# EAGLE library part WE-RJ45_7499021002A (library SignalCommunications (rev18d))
WE-RJ45 LAN Transformer Order Code 7499021002A Design THT xBase-T 10/100 Base-T Ports 1x2 Application Standard Tab Position DOWN LED (Left-Right) NO EMI Fingers No Details see: http://katalog.we-online.de/en/pbs/WE-LAN-RJ45 Created by Yingchun Shan 2016 (C) Wurth Elektronik
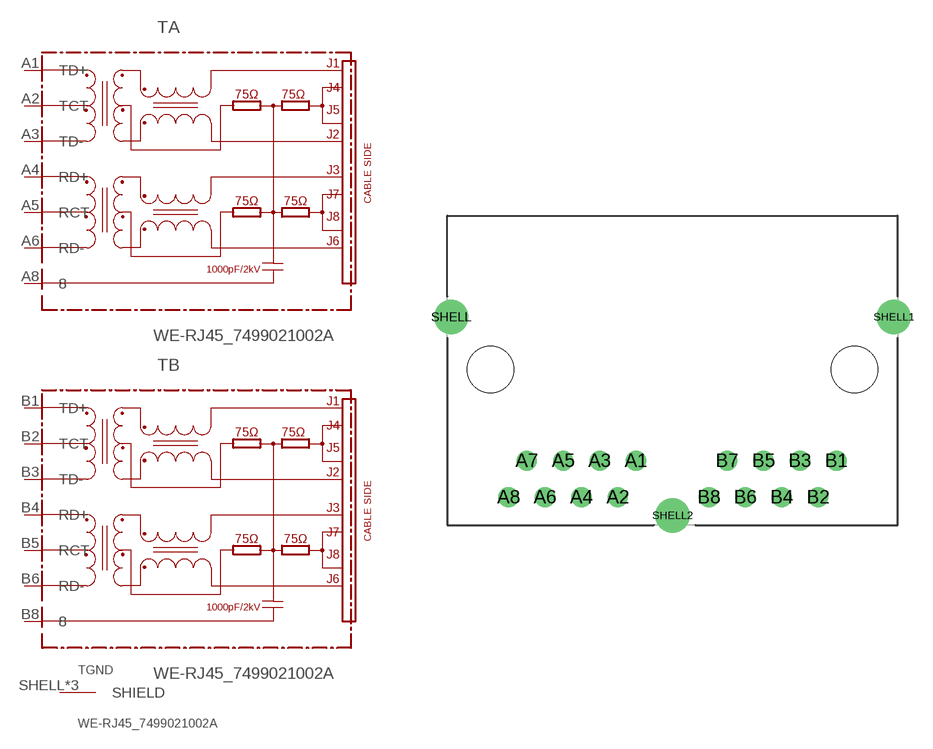
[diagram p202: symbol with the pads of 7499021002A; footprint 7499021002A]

Designator prefix T; gates A=7499021002A B=7499021002A GND=SHIELD

## WE-RJ45_7499021002A  [7499021002A]
A1  A:TD+
A2  A:TCT
A3  A:TD-
A4  A:RD+
A5  A:RCT
A6  A:RD-
A8  A:8
B1  B:TD+
B2  B:TCT
B3  B:TD-
B4  B:RD+
B5  B:RCT
B6  B:RD-
B8  B:8
SHELL  GND:SHIELD  pas
SHELL1  GND:SHIELD  pas
SHELL2  GND:SHIELD  pas

## Footprint 7499021002A (pad centres in mm)
drill 0.9: A1 -2.54,-6.35; A2 -3.81,-8.89; A3 -5.08,-6.35; A4 -6.35,-8.89; A5 -7.62,-6.35; A6 -8.89,-8.89; A7 -10.16,-6.35; A8 -11.43,-8.89; B1 11.43,-6.35; B2 10.16,-8.89; B3 8.89,-6.35; B4 7.62,-8.89; B5 6.35,-6.35; B6 5.08,-8.89; B7 3.81,-6.35; B8 2.54,-8.89
drill 1.6: SHELL -15.43,3.68; SHELL1 15.43,3.68; SHELL2 0,-10.16
hole 3.25 at -12.7,0
hole 3.25 at 12.7,0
